FUNCTION FC 30 : VOID
TITLE =BLOCK ALARM
AUTHOR : Esposito
FAMILY : EGAL_srl
NAME : ALARM
VERSION : 0.1

BEGIN
NETWORK
TITLE =ALARM TEST
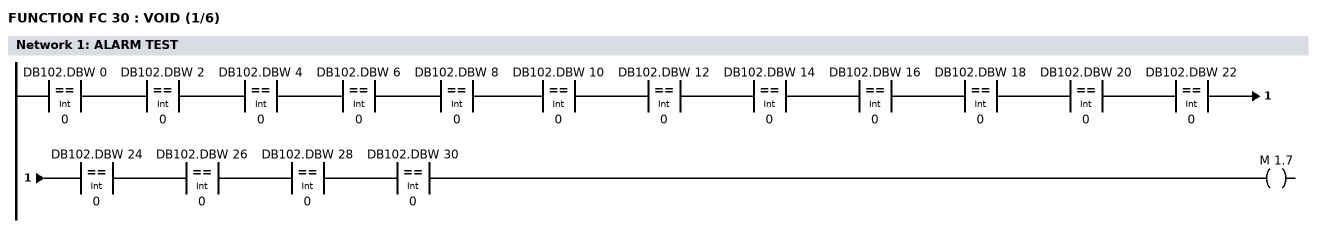
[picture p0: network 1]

      U(    ;
      L     DB102.DBW    0;
      L     0;
      ==I   ;
      )     ;
      U(    ;
      L     DB102.DBW    2;
      L     0;
      ==I   ;
      )     ;
      U(    ;
      L     DB102.DBW    4;
      L     0;
      ==I   ;
      )     ;
      U(    ;
      L     DB102.DBW    6;
      L     0;
      ==I   ;
      )     ;
      U(    ;
      L     DB102.DBW    8;
      L     0;
      ==I   ;
      )     ;
      U(    ;
      L     DB102.DBW   10;
      L     0;
      ==I   ;
      )     ;
      U(    ;
      L     DB102.DBW   12;
      L     0;
      ==I   ;
      )     ;
      U(    ;
      L     DB102.DBW   14;
      L     0;
      ==I   ;
      )     ;
      U(    ;
      L     DB102.DBW   16;
      L     0;
      ==I   ;
      )     ;
      U(    ;
      L     DB102.DBW   18;
      L     0;
      ==I   ;
      )     ;
      U(    ;
      L     DB102.DBW   20;
      L     0;
      ==I   ;
      )     ;
      U(    ;
      L     DB102.DBW   22;
      L     0;
      ==I   ;
      )     ;
      U(    ;
      L     DB102.DBW   24;
      L     0;
      ==I   ;
      )     ;
      U(    ;
      L     DB102.DBW   26;
      L     0;
      ==I   ;
      )     ;
      U(    ;
      L     DB102.DBW   28;
      L     0;
      ==I   ;
      )     ;
      U(    ;
      L     DB102.DBW   30;
      L     0;
      ==I   ;
      )     ;
      =     M      1.7;
NETWORK
TITLE =RESET ALARM ACTIVE
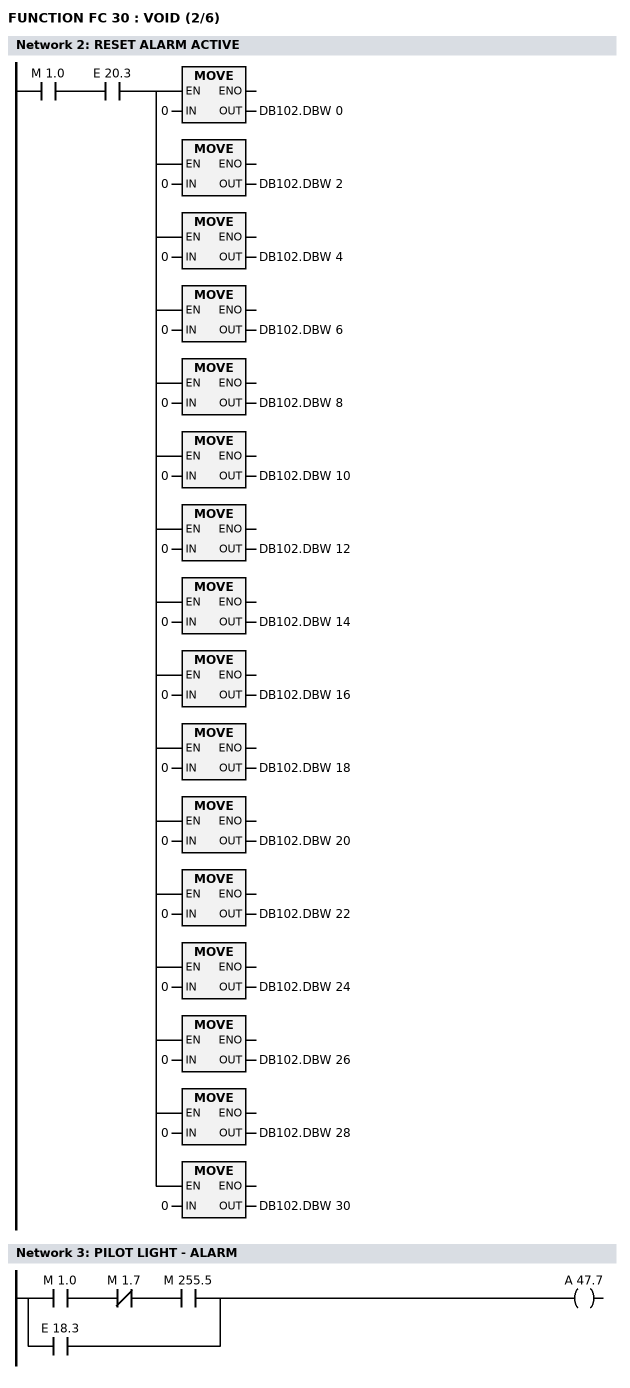
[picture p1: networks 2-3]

      U     M      1.0;
      U     E     20.3;
      =     L      0.0;
      U     L      0.0;
      SPBNB _003;
      L     0;
      T     DB102.DBW    0;
_003: NOP   0;
      U     L      0.0;
      SPBNB _009;
      L     0;
      T     DB102.DBW    2;
_009: NOP   0;
      U     L      0.0;
      SPBNB _00a;
      L     0;
      T     DB102.DBW    4;
_00a: NOP   0;
      U     L      0.0;
      SPBNB _00b;
      L     0;
      T     DB102.DBW    6;
_00b: NOP   0;
      U     L      0.0;
      SPBNB _00c;
      L     0;
      T     DB102.DBW    8;
_00c: NOP   0;
      U     L      0.0;
      SPBNB _00d;
      L     0;
      T     DB102.DBW   10;
_00d: NOP   0;
      U     L      0.0;
      SPBNB _00e;
      L     0;
      T     DB102.DBW   12;
_00e: NOP   0;
      U     L      0.0;
      SPBNB _00f;
      L     0;
      T     DB102.DBW   14;
_00f: NOP   0;
      U     L      0.0;
      SPBNB _019;
      L     0;
      T     DB102.DBW   16;
_019: NOP   0;
      U     L      0.0;
      SPBNB _01c;
      L     0;
      T     DB102.DBW   18;
_01c: NOP   0;
      U     L      0.0;
      SPBNB _01d;
      L     0;
      T     DB102.DBW   20;
_01d: NOP   0;
      U     L      0.0;
      SPBNB _01e;
      L     0;
      T     DB102.DBW   22;
_01e: NOP   0;
      U     L      0.0;
      SPBNB _021;
      L     0;
      T     DB102.DBW   24;
_021: NOP   0;
      U     L      0.0;
      SPBNB _022;
      L     0;
      T     DB102.DBW   26;
_022: NOP   0;
      U     L      0.0;
      SPBNB _023;
      L     0;
      T     DB102.DBW   28;
_023: NOP   0;
      U     L      0.0;
      SPBNB _025;
      L     0;
      T     DB102.DBW   30;
_025: NOP   0;
NETWORK
TITLE =PILOT LIGHT - ALARM

      U     M      1.0;
      UN    M      1.7;
      U     M    255.5;
      O     E     18.3;
      =     A     47.7;
NETWORK
TITLE =ALARM AUXILIARY OFF
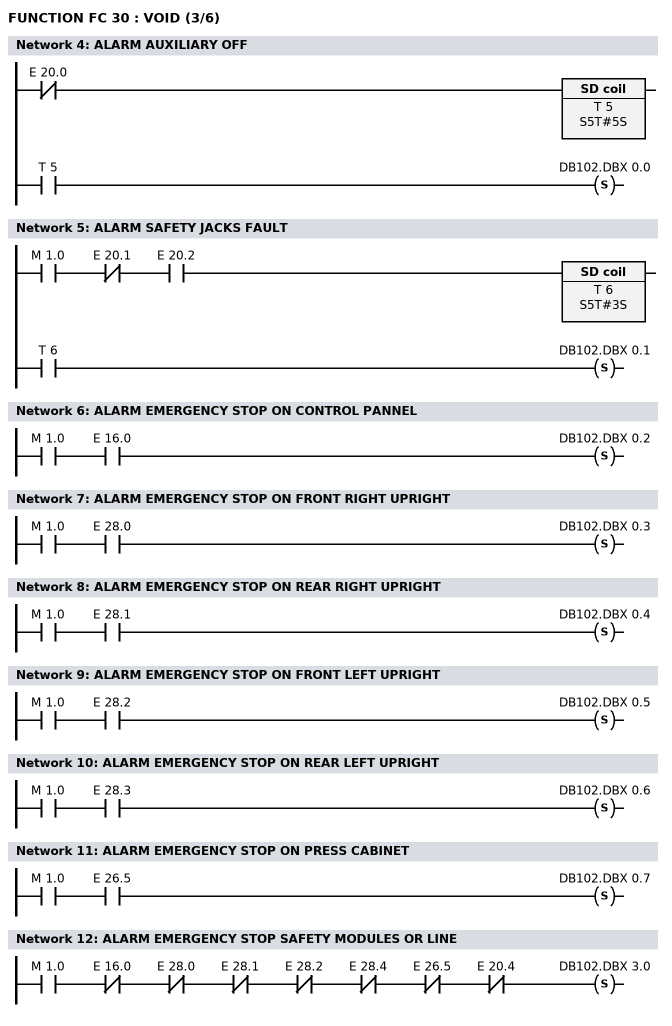
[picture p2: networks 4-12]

      UN    E     20.0;
      L     S5T#5S;
      SE    T      5;
      NOP   0;
      NOP   0;
      NOP   0;
      U     T      5;
      S     DB102.DBX    0.0;
NETWORK
TITLE =ALARM SAFETY JACKS FAULT

      U     M      1.0;
      UN    E     20.1;
      U     E     20.2;
      L     S5T#3S;
      SE    T      6;
      NOP   0;
      NOP   0;
      NOP   0;
      U     T      6;
      S     DB102.DBX    0.1;
NETWORK
TITLE =ALARM EMERGENCY STOP ON CONTROL PANNEL

      U     M      1.0;
      U     E     16.0;
      S     DB102.DBX    0.2;
NETWORK
TITLE =ALARM EMERGENCY STOP ON FRONT RIGHT UPRIGHT

      U     M      1.0;
      U     E     28.0;
      S     DB102.DBX    0.3;
NETWORK
TITLE =ALARM EMERGENCY STOP ON REAR RIGHT UPRIGHT

      U     M      1.0;
      U     E     28.1;
      S     DB102.DBX    0.4;
NETWORK
TITLE =ALARM EMERGENCY STOP ON FRONT LEFT UPRIGHT

      U     M      1.0;
      U     E     28.2;
      S     DB102.DBX    0.5;
NETWORK
TITLE =ALARM EMERGENCY STOP ON REAR LEFT UPRIGHT

      U     M      1.0;
      U     E     28.3;
      S     DB102.DBX    0.6;
NETWORK
TITLE =ALARM EMERGENCY STOP ON PRESS CABINET

      U     M      1.0;
      U     E     26.5;
      S     DB102.DBX    0.7;
NETWORK
TITLE =ALARM EMERGENCY STOP SAFETY MODULES OR LINE

      U     M      1.0;
      UN    E     16.0;
      UN    E     28.0;
      UN    E     28.1;
      UN    E     28.2;
      UN    E     28.4;
      UN    E     26.5;
      UN    E     20.4;
      S     DB102.DBX    3.0;
NETWORK
TITLE =ALARM MODE SELECTION FAULT
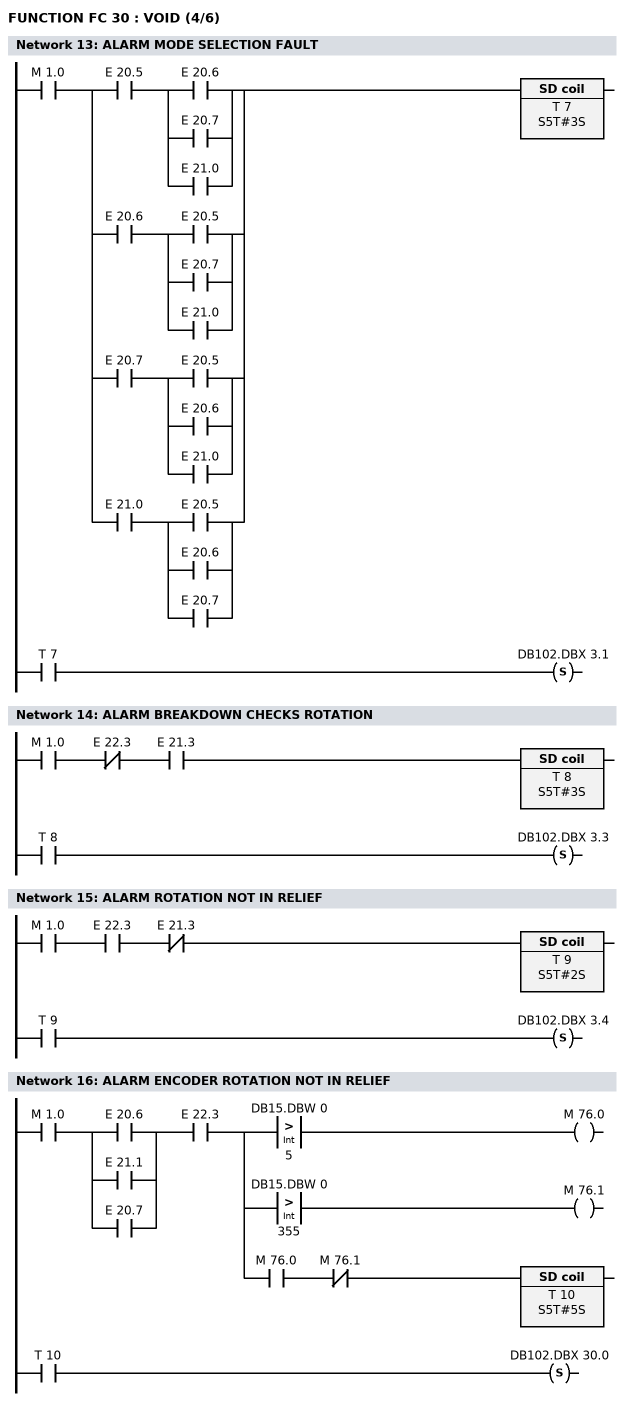
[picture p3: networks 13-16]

      U     M      1.0;
      U(    ;
      U     E     20.5;
      U(    ;
      O     E     20.6;
      O     E     20.7;
      O     E     21.0;
      )     ;
      O     ;
      U     E     20.6;
      U(    ;
      O     E     20.5;
      O     E     20.7;
      O     E     21.0;
      )     ;
      O     ;
      U     E     20.7;
      U(    ;
      O     E     20.5;
      O     E     20.6;
      O     E     21.0;
      )     ;
      O     ;
      U     E     21.0;
      U(    ;
      O     E     20.5;
      O     E     20.6;
      O     E     20.7;
      )     ;
      )     ;
      L     S5T#3S;
      SE    T      7;
      NOP   0;
      NOP   0;
      NOP   0;
      U     T      7;
      S     DB102.DBX    3.1;
NETWORK
TITLE =ALARM BREAKDOWN CHECKS ROTATION

      U     M      1.0;
      UN    E     22.3;
      U     E     21.3;
      L     S5T#3S;
      SE    T      8;
      NOP   0;
      NOP   0;
      NOP   0;
      U     T      8;
      S     DB102.DBX    3.3;
NETWORK
TITLE =ALARM ROTATION NOT IN RELIEF

      U     M      1.0;
      U     E     22.3;
      UN    E     21.3;
      L     S5T#2S;
      SE    T      9;
      NOP   0;
      NOP   0;
      NOP   0;
      U     T      9;
      S     DB102.DBX    3.4;
NETWORK
TITLE =ALARM ENCODER ROTATION NOT IN RELIEF

      U     M      1.0;
      U(    ;
      O     E     20.6;
      O     E     21.1;
      O     E     20.7;
      )     ;
      U     E     22.3;
      =     L      0.0;
      U     L      0.0;
      U(    ;
      L     DB15.DBW    0;
      L     5;
      >I    ;
      )     ;
      =     M     76.0;
      U     L      0.0;
      U(    ;
      L     DB15.DBW    0;
      L     355;
      >I    ;
      )     ;
      =     M     76.1;
      U     L      0.0;
      U     M     76.0;
      UN    M     76.1;
      L     S5T#5S;
      SE    T     10;
      NOP   0;
      NOP   0;
      NOP   0;
      U     T     10;
      S     DB102.DBX   30.0;
NETWORK
TITLE =ALARM PRESS NOT UPPER DEAD POINT
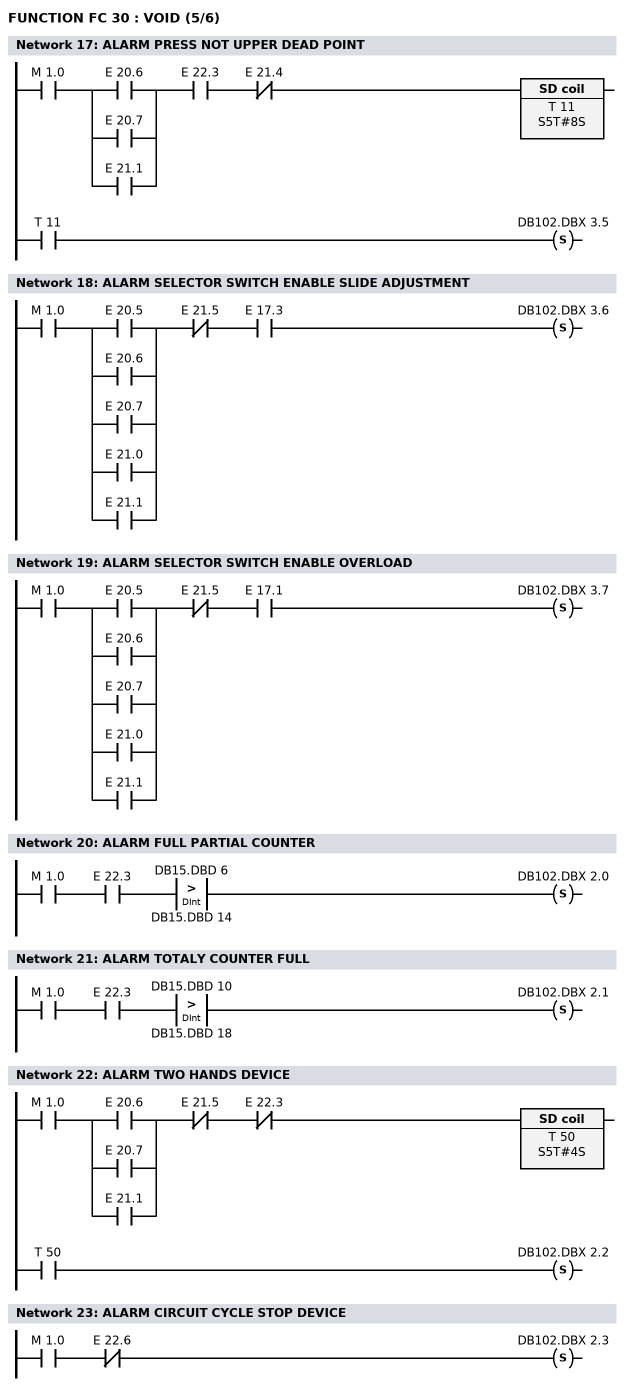
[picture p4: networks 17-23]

      U     M      1.0;
      U(    ;
      O     E     20.6;
      O     E     20.7;
      O     E     21.1;
      )     ;
      U     E     22.3;
      UN    E     21.4;
      L     S5T#8S;
      SE    T     11;
      NOP   0;
      NOP   0;
      NOP   0;
      U     T     11;
      S     DB102.DBX    3.5;
NETWORK
TITLE =ALARM SELECTOR SWITCH ENABLE SLIDE ADJUSTMENT

      U     M      1.0;
      U(    ;
      O     E     20.5;
      O     E     20.6;
      O     E     20.7;
      O     E     21.0;
      O     E     21.1;
      )     ;
      UN    E     21.5;
      U     E     17.3;
      S     DB102.DBX    3.6;
NETWORK
TITLE =ALARM SELECTOR SWITCH ENABLE OVERLOAD

      U     M      1.0;
      U(    ;
      O     E     20.5;
      O     E     20.6;
      O     E     20.7;
      O     E     21.0;
      O     E     21.1;
      )     ;
      UN    E     21.5;
      U     E     17.1;
      S     DB102.DBX    3.7;
NETWORK
TITLE =ALARM FULL PARTIAL COUNTER

      U     M      1.0;
      U     E     22.3;
      U(    ;
      L     DB15.DBD    6;
      L     DB15.DBD   14;
      >D    ;
      )     ;
      S     DB102.DBX    2.0;
NETWORK
TITLE =ALARM TOTALY COUNTER FULL

      U     M      1.0;
      U     E     22.3;
      U(    ;
      L     DB15.DBD   10;
      L     DB15.DBD   18;
      >D    ;
      )     ;
      S     DB102.DBX    2.1;
NETWORK
TITLE =ALARM TWO HANDS DEVICE

      U     M      1.0;
      U(    ;
      O     E     20.6;
      O     E     20.7;
      O     E     21.1;
      )     ;
      UN    E     21.5;
      UN    E     22.3;
      L     S5T#4S;
      SE    T     50;
      NOP   0;
      NOP   0;
      NOP   0;
      U     T     50;
      S     DB102.DBX    2.2;
NETWORK
TITLE =ALARM CIRCUIT CYCLE STOP DEVICE

      U     M      1.0;
      UN    E     22.6;
      S     DB102.DBX    2.3;
NETWORK
TITLE =ALARM LOW PRESSURE CLAMPS CIRCUIT
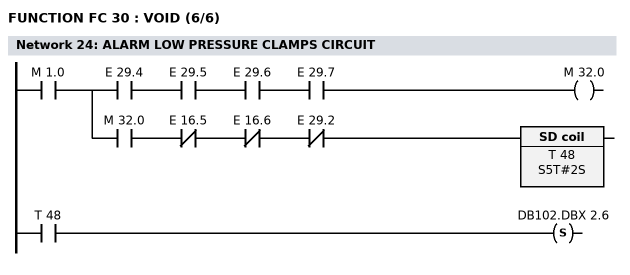
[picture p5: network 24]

      U     M      1.0;
      =     L      0.0;
      U     L      0.0;
      U     E     29.4;
      U     E     29.5;
      U     E     29.6;
      U     E     29.7;
      =     M     32.0;
      U     L      0.0;
      U     M     32.0;
      UN    E     16.5;
      UN    E     16.6;
      UN    E     29.2;
      L     S5T#2S;
      SE    T     48;
      NOP   0;
      NOP   0;
      NOP   0;
      U     T     48;
      S     DB102.DBX    2.6;
NETWORK
TITLE =ALARM CLAMPS CIRCUIT FRONT AND REAR NOT LOCK

      U     M      1.0;
      U     E     21.0;
      =     L      0.0;
      U(    ;
      U     L      0.0;
      U     E     16.5;
      S     M     12.3;
      U     M     12.4;
      R     M     12.3;
      U     M     12.3;
      )     ;
      L     S5T#30S;
      SE    T     32;
      NOP   0;
      NOP   0;
      NOP   0;
      U     T     32;
      S     DB102.DBX    2.7;
      U     L      0.0;
      U(    ;
      U     E     29.4;
      U     E     29.5;
      U     E     29.6;
      U     E     29.7;
      O     E     20.3;
      )     ;
      =     M     12.4;
NETWORK
TITLE =ALARM CLAMPS CIRCUIT FRONT AND REAR NOT UNLOCK

      U     M      1.0;
      U     E     21.0;
      =     L      0.0;
      U(    ;
      U     L      0.0;
      U     E     16.6;
      S     M     12.5;
      U     M     12.6;
      R     M     12.5;
      U     M     12.5;
      )     ;
      L     S5T#30S;
      SE    T     33;
      NOP   0;
      NOP   0;
      NOP   0;
      U     T     33;
      S     DB102.DBX    2.4;
      U     L      0.0;
      U(    ;
      U     E     30.0;
      U     E     30.1;
      U     E     30.2;
      U     E     30.3;
      O     E     20.3;
      )     ;
      =     M     12.6;
NETWORK
TITLE =ALARM THERMAL PROTECTION PUMP LUBRICATION
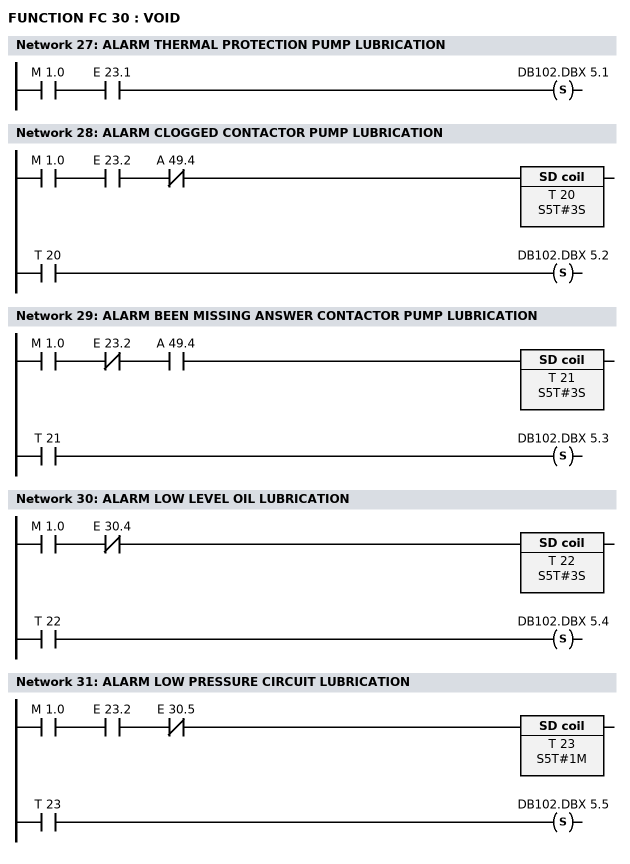
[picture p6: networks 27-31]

      U     M      1.0;
      U     E     23.1;
      S     DB102.DBX    5.1;
NETWORK
TITLE =ALARM CLOGGED CONTACTOR PUMP LUBRICATION

      U     M      1.0;
      U     E     23.2;
      UN    A     49.4;
      L     S5T#3S;
      SE    T     20;
      NOP   0;
      NOP   0;
      NOP   0;
      U     T     20;
      S     DB102.DBX    5.2;
NETWORK
TITLE =ALARM BEEN MISSING ANSWER CONTACTOR PUMP LUBRICATION

      U     M      1.0;
      UN    E     23.2;
      U     A     49.4;
      L     S5T#3S;
      SE    T     21;
      NOP   0;
      NOP   0;
      NOP   0;
      U     T     21;
      S     DB102.DBX    5.3;
NETWORK
TITLE =ALARM LOW LEVEL OIL LUBRICATION

      U     M      1.0;
      UN    E     30.4;
      L     S5T#3S;
      SE    T     22;
      NOP   0;
      NOP   0;
      NOP   0;
      U     T     22;
      S     DB102.DBX    5.4;
NETWORK
TITLE =ALARM LOW PRESSURE CIRCUIT LUBRICATION

      U     M      1.0;
      U     E     23.2;
      UN    E     30.5;
      L     S5T#1M;
      SE    T     23;
      NOP   0;
      NOP   0;
      NOP   0;
      U     T     23;
      S     DB102.DBX    5.5;
NETWORK
TITLE =ALARM LUBRICATION MONITOR TRABON

      U(    ;
      U     M      1.0;
      U     E     23.2;
      U     A     49.5;
      S     M     12.7;
      U     E     30.6;
      R     M     12.7;
      U     M     12.7;
      )     ;
      U(    ;
      O     T    100;
      O     M     42.0;
      )     ;
      L     S5T#1M;
      SE    T     34;
      NOP   0;
      NOP   0;
      NOP   0;
      U     T     34;
      S     DB102.DBX    5.6;
NETWORK
TITLE =ALARM LOW OIL LEVEL OVERLOAD
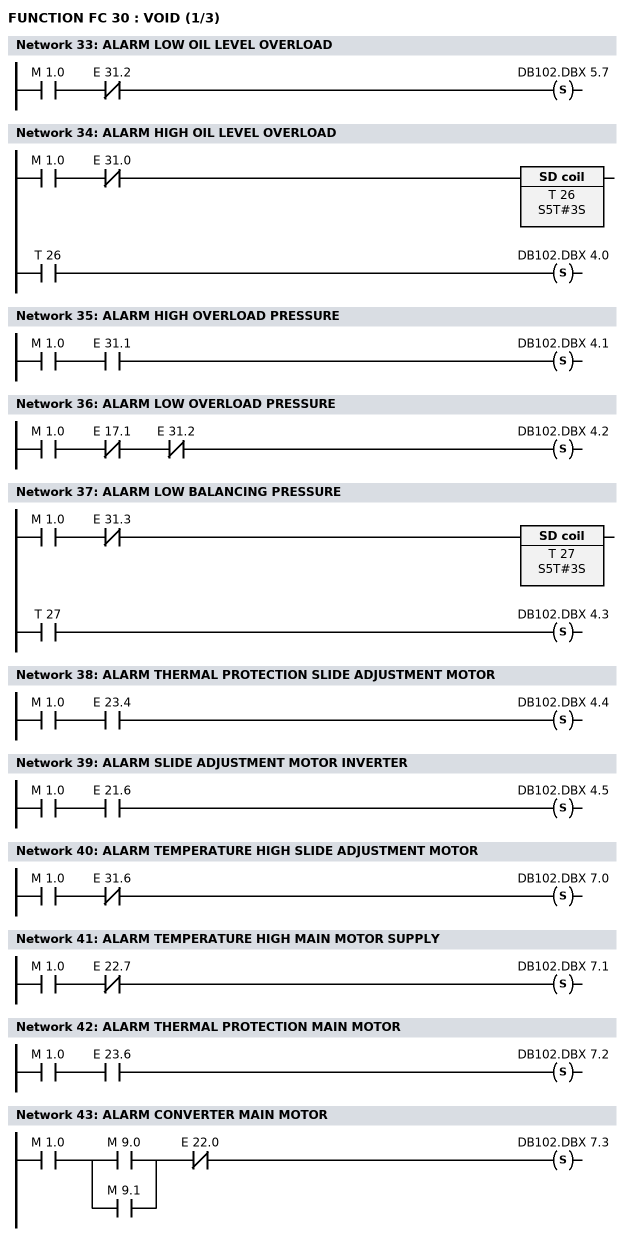
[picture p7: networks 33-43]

      U     M      1.0;
      UN    E     31.2;
      S     DB102.DBX    5.7;
NETWORK
TITLE =ALARM HIGH OIL LEVEL OVERLOAD

      U     M      1.0;
      UN    E     31.0;
      L     S5T#3S;
      SE    T     26;
      NOP   0;
      NOP   0;
      NOP   0;
      U     T     26;
      S     DB102.DBX    4.0;
NETWORK
TITLE =ALARM HIGH OVERLOAD PRESSURE

      U     M      1.0;
      U     E     31.1;
      S     DB102.DBX    4.1;
NETWORK
TITLE =ALARM LOW OVERLOAD PRESSURE

      U     M      1.0;
      UN    E     17.1;
      UN    E     31.2;
      S     DB102.DBX    4.2;
NETWORK
TITLE =ALARM LOW BALANCING PRESSURE

      U     M      1.0;
      UN    E     31.3;
      L     S5T#3S;
      SE    T     27;
      NOP   0;
      NOP   0;
      NOP   0;
      U     T     27;
      S     DB102.DBX    4.3;
NETWORK
TITLE =ALARM THERMAL PROTECTION SLIDE ADJUSTMENT MOTOR

      U     M      1.0;
      U     E     23.4;
      S     DB102.DBX    4.4;
NETWORK
TITLE =ALARM SLIDE ADJUSTMENT MOTOR INVERTER

      U     M      1.0;
      U     E     21.6;
      S     DB102.DBX    4.5;
NETWORK
TITLE =ALARM TEMPERATURE HIGH SLIDE ADJUSTMENT MOTOR

      U     M      1.0;
      UN    E     31.6;
      S     DB102.DBX    7.0;
NETWORK
TITLE =ALARM TEMPERATURE HIGH MAIN MOTOR SUPPLY

      U     M      1.0;
      UN    E     22.7;
      S     DB102.DBX    7.1;
NETWORK
TITLE =ALARM THERMAL PROTECTION MAIN MOTOR

      U     M      1.0;
      U     E     23.6;
      S     DB102.DBX    7.2;
NETWORK
TITLE =ALARM CONVERTER MAIN MOTOR

      U     M      1.0;
      U(    ;
      O     M      9.0;
      O     M      9.1;
      )     ;
      UN    E     22.0;
      S     DB102.DBX    7.3;
NETWORK
TITLE =ALARM LINE CONTACTOR MAIN MOTOR
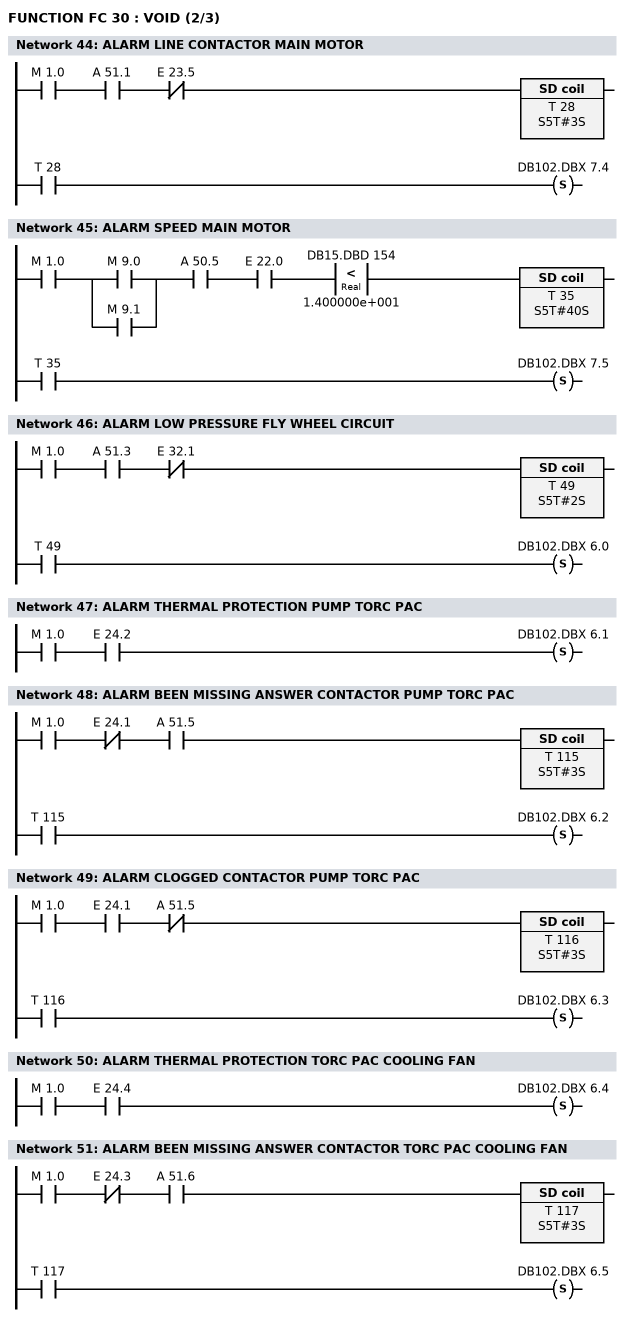
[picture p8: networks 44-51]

      U     M      1.0;
      U     A     51.1;
      UN    E     23.5;
      L     S5T#3S;
      SE    T     28;
      NOP   0;
      NOP   0;
      NOP   0;
      U     T     28;
      S     DB102.DBX    7.4;
NETWORK
TITLE =ALARM SPEED MAIN MOTOR

      U     M      1.0;
      U(    ;
      O     M      9.0;
      O     M      9.1;
      )     ;
      U     A     50.5;
      U     E     22.0;
      U(    ;
      L     DB15.DBD  154;
      L     1.400000e+001;
      <R    ;
      )     ;
      L     S5T#40S;
      SE    T     35;
      NOP   0;
      NOP   0;
      NOP   0;
      U     T     35;
      S     DB102.DBX    7.5;
NETWORK
TITLE =ALARM LOW PRESSURE FLY WHEEL CIRCUIT

      U     M      1.0;
      U     A     51.3;
      UN    E     32.1;
      L     S5T#2S;
      SE    T     49;
      NOP   0;
      NOP   0;
      NOP   0;
      U     T     49;
      S     DB102.DBX    6.0;
NETWORK
TITLE =ALARM THERMAL PROTECTION PUMP TORC PAC

      U     M      1.0;
      U     E     24.2;
      S     DB102.DBX    6.1;
NETWORK
TITLE =ALARM BEEN MISSING ANSWER CONTACTOR PUMP TORC PAC

      U     M      1.0;
      UN    E     24.1;
      U     A     51.5;
      L     S5T#3S;
      SE    T    115;
      NOP   0;
      NOP   0;
      NOP   0;
      U     T    115;
      S     DB102.DBX    6.2;
NETWORK
TITLE =ALARM CLOGGED CONTACTOR PUMP TORC PAC

      U     M      1.0;
      U     E     24.1;
      UN    A     51.5;
      L     S5T#3S;
      SE    T    116;
      NOP   0;
      NOP   0;
      NOP   0;
      U     T    116;
      S     DB102.DBX    6.3;
NETWORK
TITLE =ALARM THERMAL PROTECTION TORC PAC COOLING FAN

      U     M      1.0;
      U     E     24.4;
      S     DB102.DBX    6.4;
NETWORK
TITLE =ALARM BEEN MISSING ANSWER CONTACTOR TORC PAC COOLING FAN

      U     M      1.0;
      UN    E     24.3;
      U     A     51.6;
      L     S5T#3S;
      SE    T    117;
      NOP   0;
      NOP   0;
      NOP   0;
      U     T    117;
      S     DB102.DBX    6.5;
NETWORK
TITLE =ALARM CLOGGED CONTACTOR TORC PAC COOLING FAN
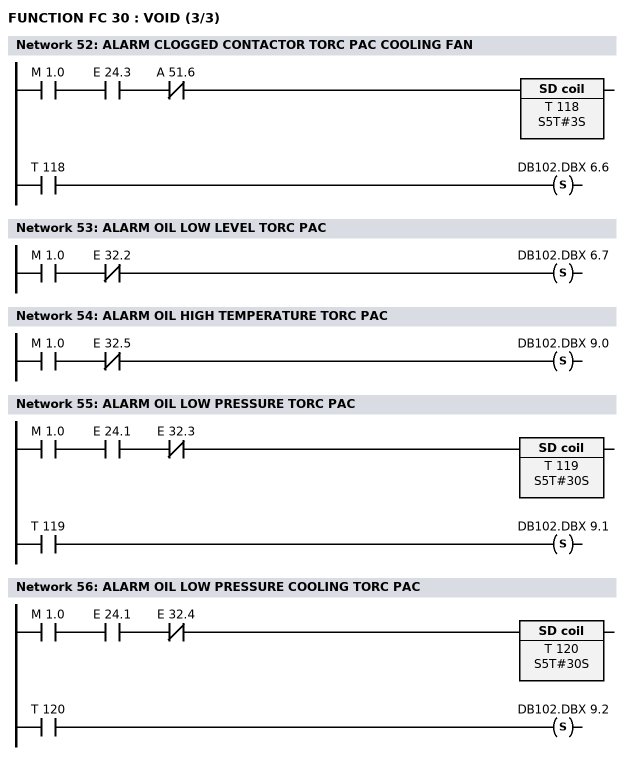
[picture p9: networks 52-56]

      U     M      1.0;
      U     E     24.3;
      UN    A     51.6;
      L     S5T#3S;
      SE    T    118;
      NOP   0;
      NOP   0;
      NOP   0;
      U     T    118;
      S     DB102.DBX    6.6;
NETWORK
TITLE =ALARM OIL LOW LEVEL TORC PAC

      U     M      1.0;
      UN    E     32.2;
      S     DB102.DBX    6.7;
NETWORK
TITLE =ALARM OIL HIGH TEMPERATURE TORC PAC

      U     M      1.0;
      UN    E     32.5;
      S     DB102.DBX    9.0;
NETWORK
TITLE =ALARM OIL LOW PRESSURE TORC PAC

      U     M      1.0;
      U     E     24.1;
      UN    E     32.3;
      L     S5T#30S;
      SE    T    119;
      NOP   0;
      NOP   0;
      NOP   0;
      U     T    119;
      S     DB102.DBX    9.1;
NETWORK
TITLE =ALARM OIL LOW PRESSURE COOLING TORC PAC

      U     M      1.0;
      U     E     24.1;
      UN    E     32.4;
      L     S5T#30S;
      SE    T    120;
      NOP   0;
      NOP   0;
      NOP   0;
      U     T    120;
      S     DB102.DBX    9.2;
NETWORK
TITLE =ALARM DOUBLE STROKE CONTROL

      U(    ;
      U     M      1.0;
      U(    ;
      O     E     20.6;
      O     E     20.7;
      O     E     21.1;
      )     ;
      U     E     22.2;
      L     S5T#4S;
      SE    T     37;
      NOP   0;
      NOP   0;
      NOP   0;
      U     T     37;
      )     ;
      FP    M     10.7;
      S     DB102.DBX    9.3;
NETWORK
TITLE =ALARM CLUTCH BRAKE UNIT CONTROL NOT OK
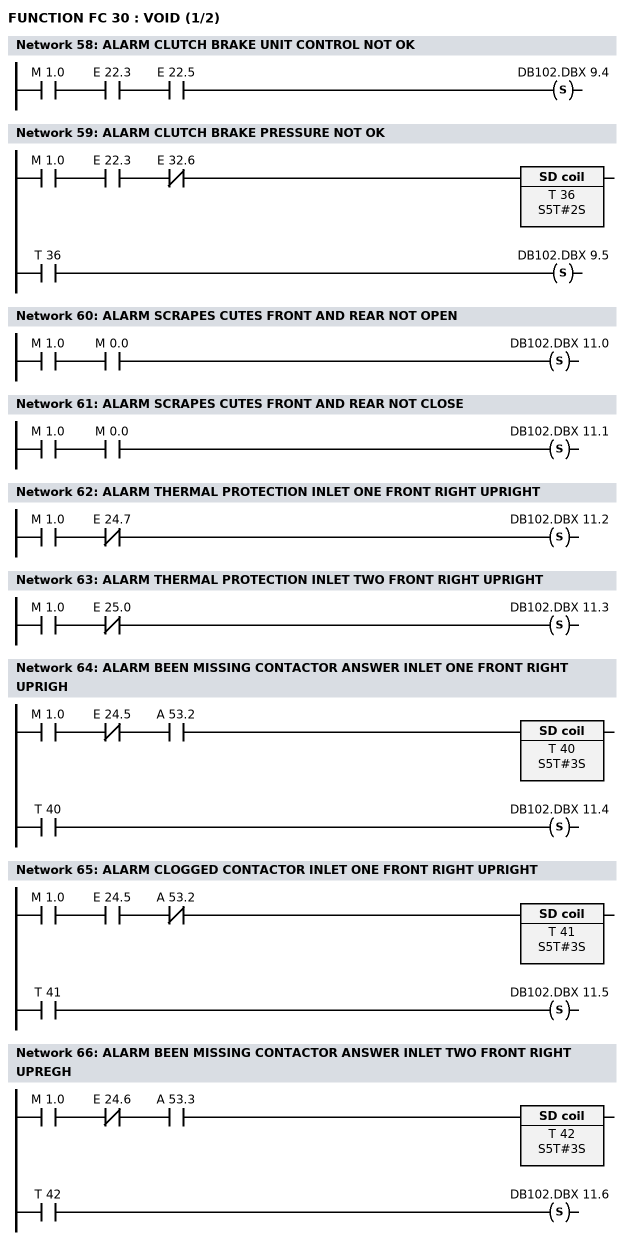
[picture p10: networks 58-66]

      U     M      1.0;
      U     E     22.3;
      U     E     22.5;
      S     DB102.DBX    9.4;
NETWORK
TITLE =ALARM CLUTCH BRAKE PRESSURE NOT OK

      U     M      1.0;
      U     E     22.3;
      UN    E     32.6;
      L     S5T#2S;
      SE    T     36;
      NOP   0;
      NOP   0;
      NOP   0;
      U     T     36;
      S     DB102.DBX    9.5;
NETWORK
TITLE =ALARM SCRAPES CUTES FRONT AND REAR NOT OPEN

      U     M      1.0;
      U     M      0.0;
      S     DB102.DBX   11.0;
NETWORK
TITLE =ALARM SCRAPES CUTES FRONT AND REAR NOT CLOSE

      U     M      1.0;
      U     M      0.0;
      S     DB102.DBX   11.1;
NETWORK
TITLE =ALARM THERMAL PROTECTION INLET ONE FRONT RIGHT UPRIGHT

      U     M      1.0;
      UN    E     24.7;
      S     DB102.DBX   11.2;
NETWORK
TITLE =ALARM THERMAL PROTECTION INLET TWO FRONT RIGHT UPRIGHT

      U     M      1.0;
      UN    E     25.0;
      S     DB102.DBX   11.3;
NETWORK
TITLE =ALARM BEEN MISSING CONTACTOR ANSWER INLET ONE FRONT RIGHT UPRIGH

      U     M      1.0;
      UN    E     24.5;
      U     A     53.2;
      L     S5T#3S;
      SE    T     40;
      NOP   0;
      NOP   0;
      NOP   0;
      U     T     40;
      S     DB102.DBX   11.4;
NETWORK
TITLE =ALARM CLOGGED CONTACTOR INLET ONE FRONT RIGHT UPRIGHT

      U     M      1.0;
      U     E     24.5;
      UN    A     53.2;
      L     S5T#3S;
      SE    T     41;
      NOP   0;
      NOP   0;
      NOP   0;
      U     T     41;
      S     DB102.DBX   11.5;
NETWORK
TITLE =ALARM BEEN MISSING CONTACTOR ANSWER INLET TWO FRONT RIGHT UPREGH

      U     M      1.0;
      UN    E     24.6;
      U     A     53.3;
      L     S5T#3S;
      SE    T     42;
      NOP   0;
      NOP   0;
      NOP   0;
      U     T     42;
      S     DB102.DBX   11.6;
NETWORK
TITLE =ALARM CLOGGED CONTACTOR INLET TWO FRONT RIGHT UPRIGHT
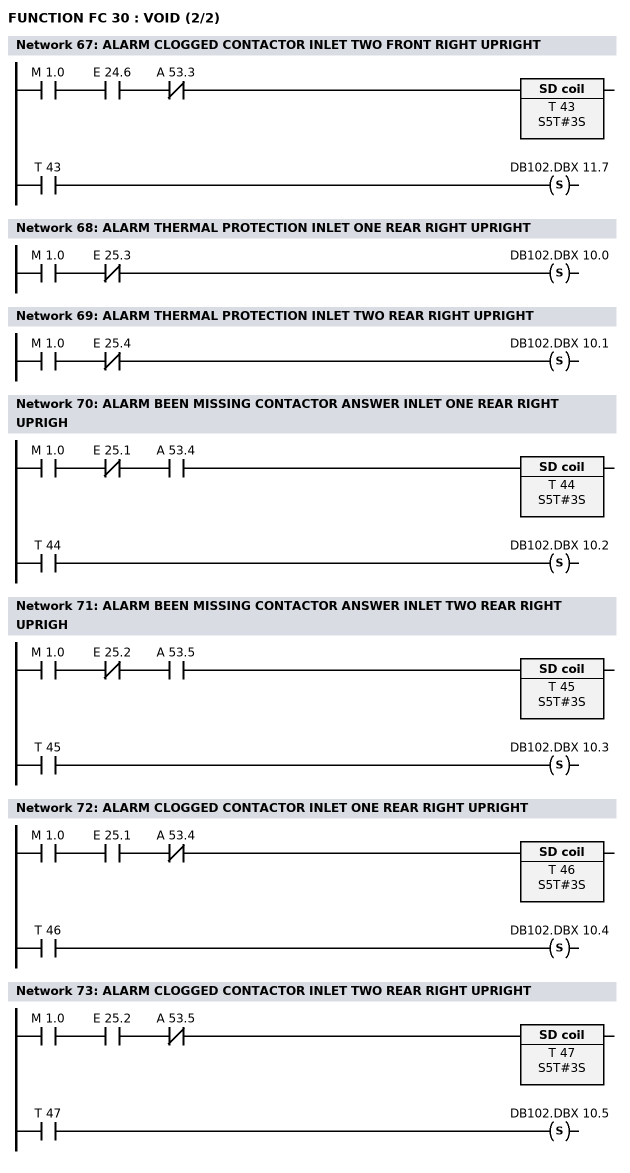
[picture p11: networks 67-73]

      U     M      1.0;
      U     E     24.6;
      UN    A     53.3;
      L     S5T#3S;
      SE    T     43;
      NOP   0;
      NOP   0;
      NOP   0;
      U     T     43;
      S     DB102.DBX   11.7;
NETWORK
TITLE =ALARM THERMAL PROTECTION INLET ONE REAR RIGHT UPRIGHT

      U     M      1.0;
      UN    E     25.3;
      S     DB102.DBX   10.0;
NETWORK
TITLE =ALARM THERMAL PROTECTION INLET TWO REAR RIGHT UPRIGHT

      U     M      1.0;
      UN    E     25.4;
      S     DB102.DBX   10.1;
NETWORK
TITLE =ALARM BEEN MISSING CONTACTOR ANSWER INLET ONE REAR RIGHT UPRIGH

      U     M      1.0;
      UN    E     25.1;
      U     A     53.4;
      L     S5T#3S;
      SE    T     44;
      NOP   0;
      NOP   0;
      NOP   0;
      U     T     44;
      S     DB102.DBX   10.2;
NETWORK
TITLE =ALARM BEEN MISSING CONTACTOR ANSWER INLET TWO REAR RIGHT UPRIGH

      U     M      1.0;
      UN    E     25.2;
      U     A     53.5;
      L     S5T#3S;
      SE    T     45;
      NOP   0;
      NOP   0;
      NOP   0;
      U     T     45;
      S     DB102.DBX   10.3;
NETWORK
TITLE =ALARM CLOGGED CONTACTOR INLET ONE REAR RIGHT UPRIGHT

      U     M      1.0;
      U     E     25.1;
      UN    A     53.4;
      L     S5T#3S;
      SE    T     46;
      NOP   0;
      NOP   0;
      NOP   0;
      U     T     46;
      S     DB102.DBX   10.4;
NETWORK
TITLE =ALARM CLOGGED CONTACTOR INLET TWO REAR RIGHT UPRIGHT

      U     M      1.0;
      U     E     25.2;
      UN    A     53.5;
      L     S5T#3S;
      SE    T     47;
      NOP   0;
      NOP   0;
      NOP   0;
      U     T     47;
      S     DB102.DBX   10.5;
NETWORK
TITLE =ALARM EMERGENCY STOP OPERATORPANEL BLACKCARTS

      U     M      1.0;
      L     DB4.DBW   24;
      L     W#16#1;
      ==I   ;
      =     DB102.DBX   13.0;
NETWORK
TITLE =ALARM EMERGENCY STOP GATE BLANCKCARTS 1

      U     M      1.0;
      L     DB4.DBW   24;
      L     W#16#2;
      ==I   ;
      =     DB102.DBX   13.1;
NETWORK
TITLE =ALARM EMERGENCY STOP GATE BLANCKCARTS 2

      U     M      1.0;
      L     DB4.DBW   24;
      L     W#16#3;
      ==I   ;
      =     DB102.DBX   13.2;
NETWORK
TITLE =ALARM EMERGENCY STOP AUXILIARY ROBOT CABINET 1

      U     M      1.0;
      L     DB4.DBW   24;
      L     W#16#4;
      ==I   ;
      =     DB102.DBX   13.3;
NETWORK
TITLE =ALARM EMERGENCY STOP AUXILIARY ROBOT CABINET 2

      U     M      1.0;
      L     DB4.DBW   24;
      L     W#16#5;
      ==I   ;
      =     DB102.DBX   13.4;
NETWORK
TITLE =ALARM EMERGENCY STOP GATE ROBOT 1

      U     M      1.0;
      L     DB4.DBW   24;
      L     W#16#6;
      ==I   ;
      =     DB102.DBX   13.5;
NETWORK
TITLE =ALARM EMERGENCY STOP GATE ROBOT 2

      U     M      1.0;
      L     DB4.DBW   24;
      L     W#16#7;
      ==I   ;
      =     DB102.DBX   13.6;
NETWORK
TITLE =ALARM EMERGENCY STOP HANDTERMINAL CENTERING TABLE

      U     M      1.0;
      L     DB4.DBW   24;
      L     W#16#8;
      ==I   ;
      =     DB102.DBX   13.7;
NETWORK
TITLE =ALARM GATE 1 NOT CLOSED AND LOCKED

      U     M      1.0;
      UN    E     21.0;
      UN    E     20.5;
      L     DB4.DBW   24;
      L     W#16#21;
      ==I   ;
      =     DB102.DBX   12.0;
NETWORK
TITLE =ALARM GATE 2 NOT CLOSED AND LOCKED

      U     M      1.0;
      UN    E     21.0;
      UN    E     20.5;
      L     DB4.DBW   24;
      L     W#16#A;
      ==I   ;
      =     DB102.DBX   12.1;
NETWORK
TITLE =ALARM GATE 3 NOT CLOSED AND LOCKED

      U     M      1.0;
      UN    E     21.0;
      UN    E     20.5;
      L     DB4.DBW   24;
      L     W#16#B;
      ==I   ;
      =     DB102.DBX   12.2;
NETWORK
TITLE =ALARM GATE 4 NOT CLOSED AND LOCKED

      U     M      1.0;
      UN    E     21.0;
      UN    E     20.5;
      L     DB4.DBW   24;
      L     W#16#C;
      ==I   ;
      =     DB102.DBX   12.3;
NETWORK
TITLE =ALARM GATE 5 NOT CLOSED AND LOCKED

      U     M      1.0;
      UN    E     21.0;
      UN    E     20.5;
      L     DB4.DBW   24;
      L     W#16#D;
      ==I   ;
      =     DB102.DBX   12.4;
NETWORK
TITLE =ALARM GATE 6 NOT CLOSED AND LOCKED

      U     M      1.0;
      UN    E     21.0;
      UN    E     20.5;
      L     DB4.DBW   24;
      L     W#16#E;
      ==I   ;
      =     DB102.DBX   12.5;
NETWORK
TITLE =ALARM GATE 7 NOT CLOSED AND LOCKED

      U     M      1.0;
      UN    E     21.0;
      UN    E     20.5;
      L     DB4.DBW   24;
      L     W#16#F;
      ==I   ;
      =     DB102.DBX   12.6;
NETWORK
TITLE =ALARM LIGHTCURTAIN BLANCKCARTS

      U     M      1.0;
      L     DB4.DBW   24;
      L     W#16#10;
      ==I   ;
      =     DB102.DBX   12.7;
NETWORK
TITLE =ALARM OVERLOAD MOTORS AUXILIARY EQUIPMENT

      U     M      1.0;
      L     DB4.DBW   24;
      L     W#16#11;
      ==I   ;
      =     DB102.DBX   15.0;
NETWORK
TITLE =ALARM OVERLOAD POWERSUPPLY AUXILIARY EQUIPMENT

      U     M      1.0;
      L     DB4.DBW   24;
      L     W#16#12;
      ==I   ;
      U     M      0.0;
      =     DB102.DBX   15.1;
NETWORK
TITLE =ALARM OVERLOAD POWERSUPPLY OPERATORPANEL BLANCKCARTS

      U     M      1.0;
      L     DB4.DBW   24;
      L     W#16#13;
      ==I   ;
      =     DB102.DBX   15.2;
NETWORK
TITLE =ALARM CURRENT CONTROL RELAY CONVOYER
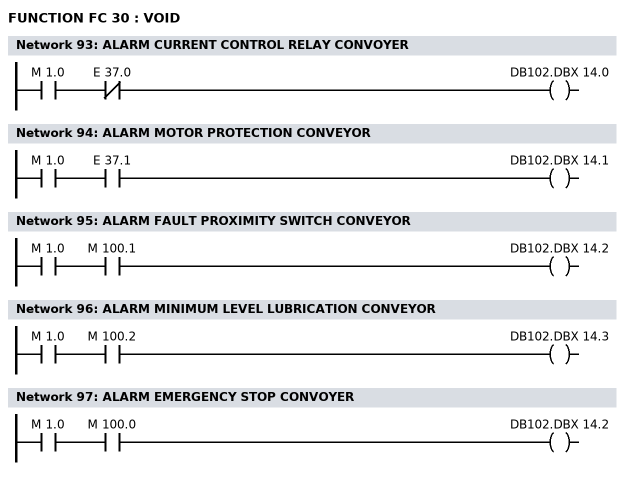
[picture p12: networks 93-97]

      U     M      1.0;
      UN    E     37.0;
      =     DB102.DBX   14.0;
NETWORK
TITLE =ALARM MOTOR PROTECTION CONVEYOR

      U     M      1.0;
      U     E     37.1;
      =     DB102.DBX   14.1;
NETWORK
TITLE =ALARM FAULT PROXIMITY SWITCH CONVEYOR

      U     M      1.0;
      U     M    100.1;
      =     DB102.DBX   14.2;
NETWORK
TITLE =ALARM MINIMUM LEVEL LUBRICATION CONVEYOR

      U     M      1.0;
      U     M    100.2;
      =     DB102.DBX   14.3;
NETWORK
TITLE =ALARM EMERGENCY STOP CONVOYER

      U     M      1.0;
      U     M    100.0;
      =     DB102.DBX   14.2;
END_FUNCTION

